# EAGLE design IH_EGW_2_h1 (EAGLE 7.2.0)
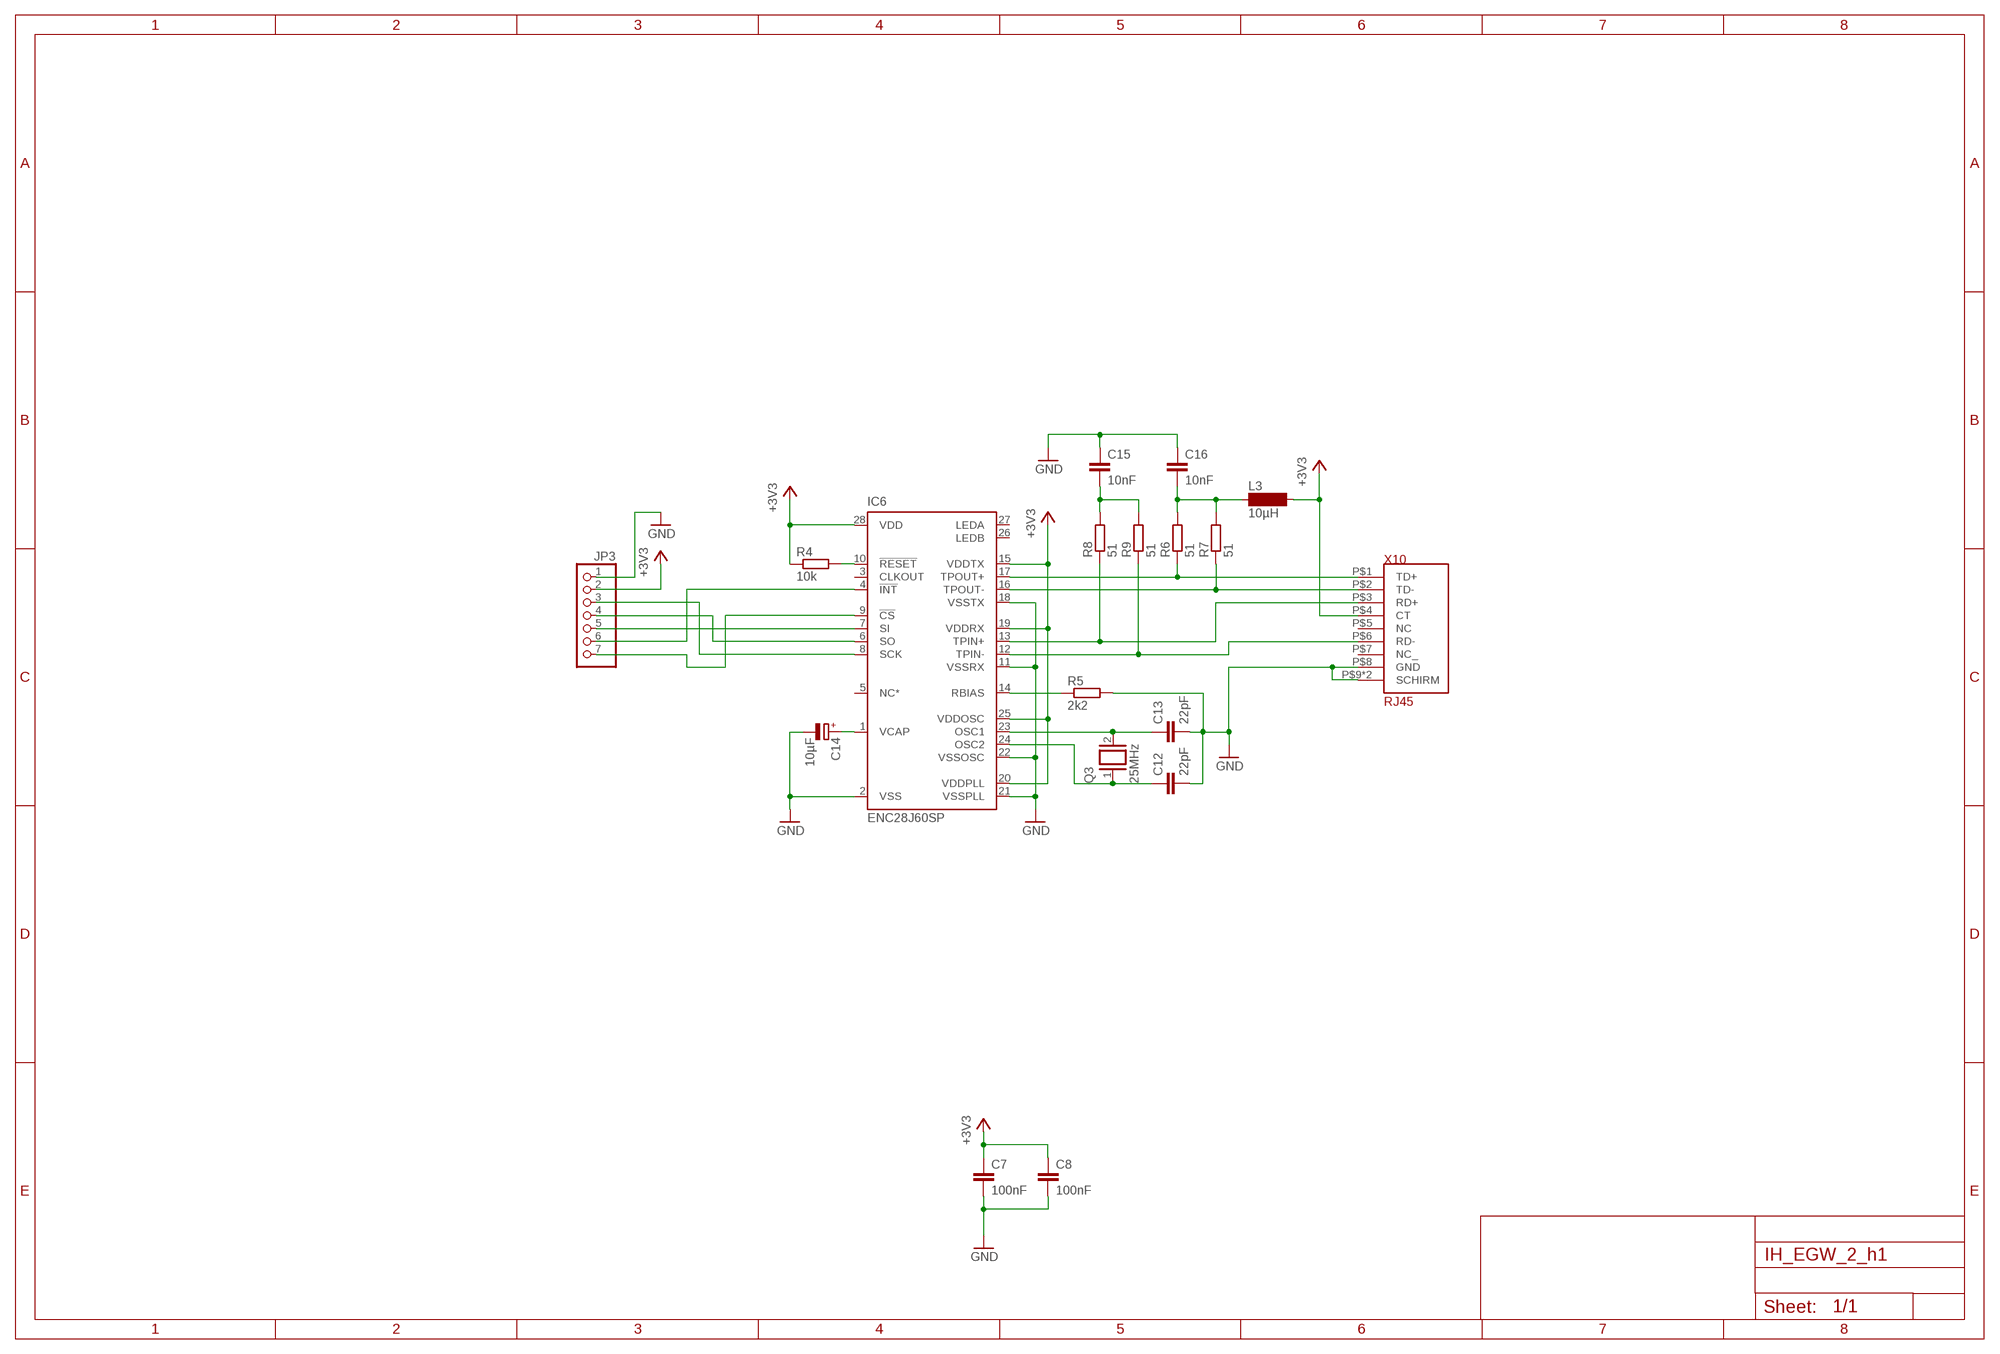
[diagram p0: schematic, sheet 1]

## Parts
C7  100nF  C-EUC0805  [C0805]
C8  100nF  C-EUC0805  [C0805]
C12  22pF  C-EUC0805  [C0805]
C13  22pF  C-EUC0805  [C0805]
C14  10µF  CPOL-EUE2-5  [E2-5]
C15  10nF  C-EUC0805  [C0805]
C16  10nF  C-EUC0805  [C0805]
IC6  ENC28J60SP  [DIL28-3]
JP3  PINHD-1X7  [1X07]
L3  10µH  SD12-1000  [SD12_1000]
Q3  25MHz  XTAL/S  [QS]
R4  10k  R-EU_R0805  [R0805]
R5  2k2  R-EU_R0805  [R0805]
R6  51  R-EU_M0805  [M0805]
R7  51  R-EU_M0805  [M0805]
R8  51  R-EU_M0805  [M0805]
R9  51  R-EU_M0805  [M0805]
X10  RJ45  [RJ45_LIEGEND]

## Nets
+3V3: C7.1 C8.1 IC6.15(VDDTX) IC6.19(VDDRX) IC6.20(VDDPLL) IC6.25(VDDOSC) IC6.28(VDD) JP3.2 L3.2 R4.1 X10.P$4(CT)
GND: C7.2 C8.2 C12.2 C13.2 C14.- C15.1 C16.1 IC6.2(VSS) IC6.11(VSSRX) IC6.18(VSSTX) IC6.21(VSSPLL) IC6.22(VSSOSC) JP3.1 R5.2 X10.P$8(GND) X10.P$9(SCHIRM) X10.P$10(SCHIRM)
INT_E: IC6.4(!INT) JP3.6
MISO: IC6.6(SO) JP3.4
N$1: IC6.7(SI) JP3.5
N$5: IC6.14(RBIAS) R5.1
N$6: C14.+ IC6.1(VCAP)
N$9: IC6.13(TPIN+) R8.1 X10.P$3(RD+)
N$10: IC6.12(TPIN-) R9.1 X10.P$6(RD-)
N$11: IC6.17(TPOUT+) R6.1 X10.P$1(TD+)
N$12: IC6.16(TPOUT-) R7.1 X10.P$2(TD-)
N$13: C15.2 R8.2 R9.2
N$14: C16.2 L3.1 R6.2 R7.2
N$28: C13.1 IC6.23(OSC1) Q3.2
N$29: C12.1 IC6.24(OSC2) Q3.1
N$30: IC6.10(!RESET) R4.2
SCK: IC6.8(SCK) JP3.3
SS: IC6.9(!CS) JP3.7
Unconnected: IC6.3(CLKOUT) IC6.5(NC*) IC6.26(LEDB) IC6.27(LEDA) X10.P$5(NC) X10.P$7(NC_)

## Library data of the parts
C7 C8 C12 C13 C15 C16 = rcl:C-EU: CAPACITOR, European symbol
C14 = rcl:CPOL-EU: POLARIZED CAPACITOR, European symbol
IC6 = microchip:ENC28J60: Stand-Alone Ethernet Controller with SPI Interface Source: http://ww1.microchip.com/downloads/en/DeviceDoc/39662c.pdf; MF: MICROCHIP; MPN: ENC28J60/SP; OC_FARNELL: 1084619; OC_NEWARK: 96K3661
JP3 = pinhead:PINHD-1X7: PIN HEADER
L3 = inductor-neosid:SD12: INDUCTOR; OC_FARNELL: unknown; OC_NEWARK: unknown
Q3 = special:XTAL/S: CRYSTAL
R4-R9 = resistor:R-EU_: RESISTOR, European symbol
X10 = RJ45:RJ45

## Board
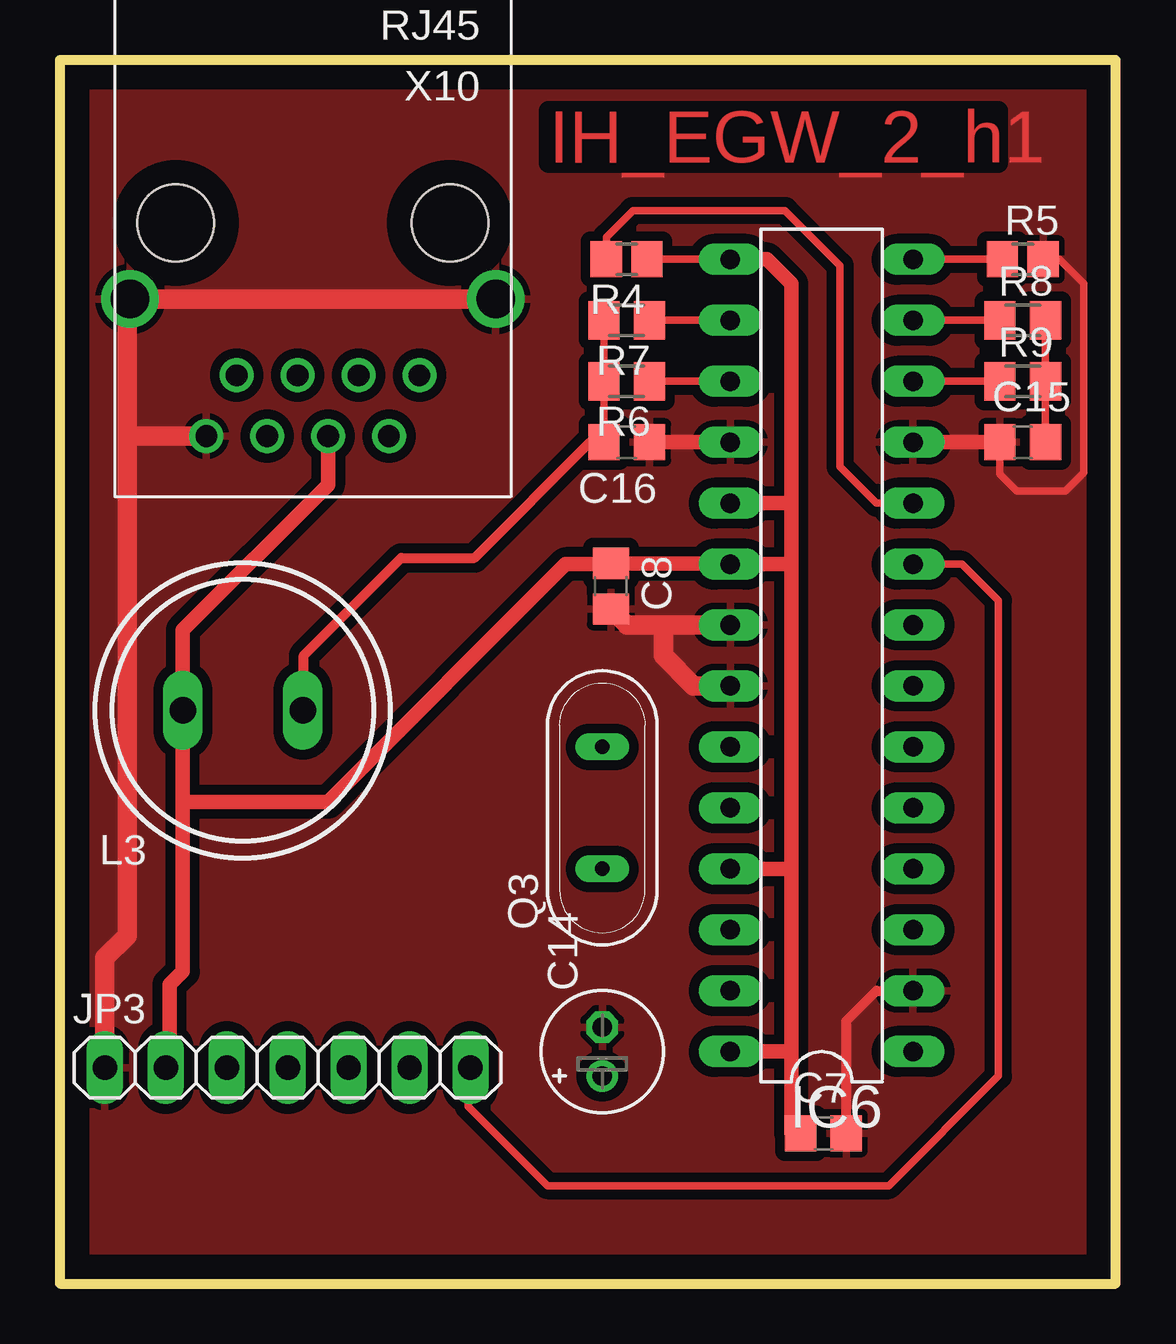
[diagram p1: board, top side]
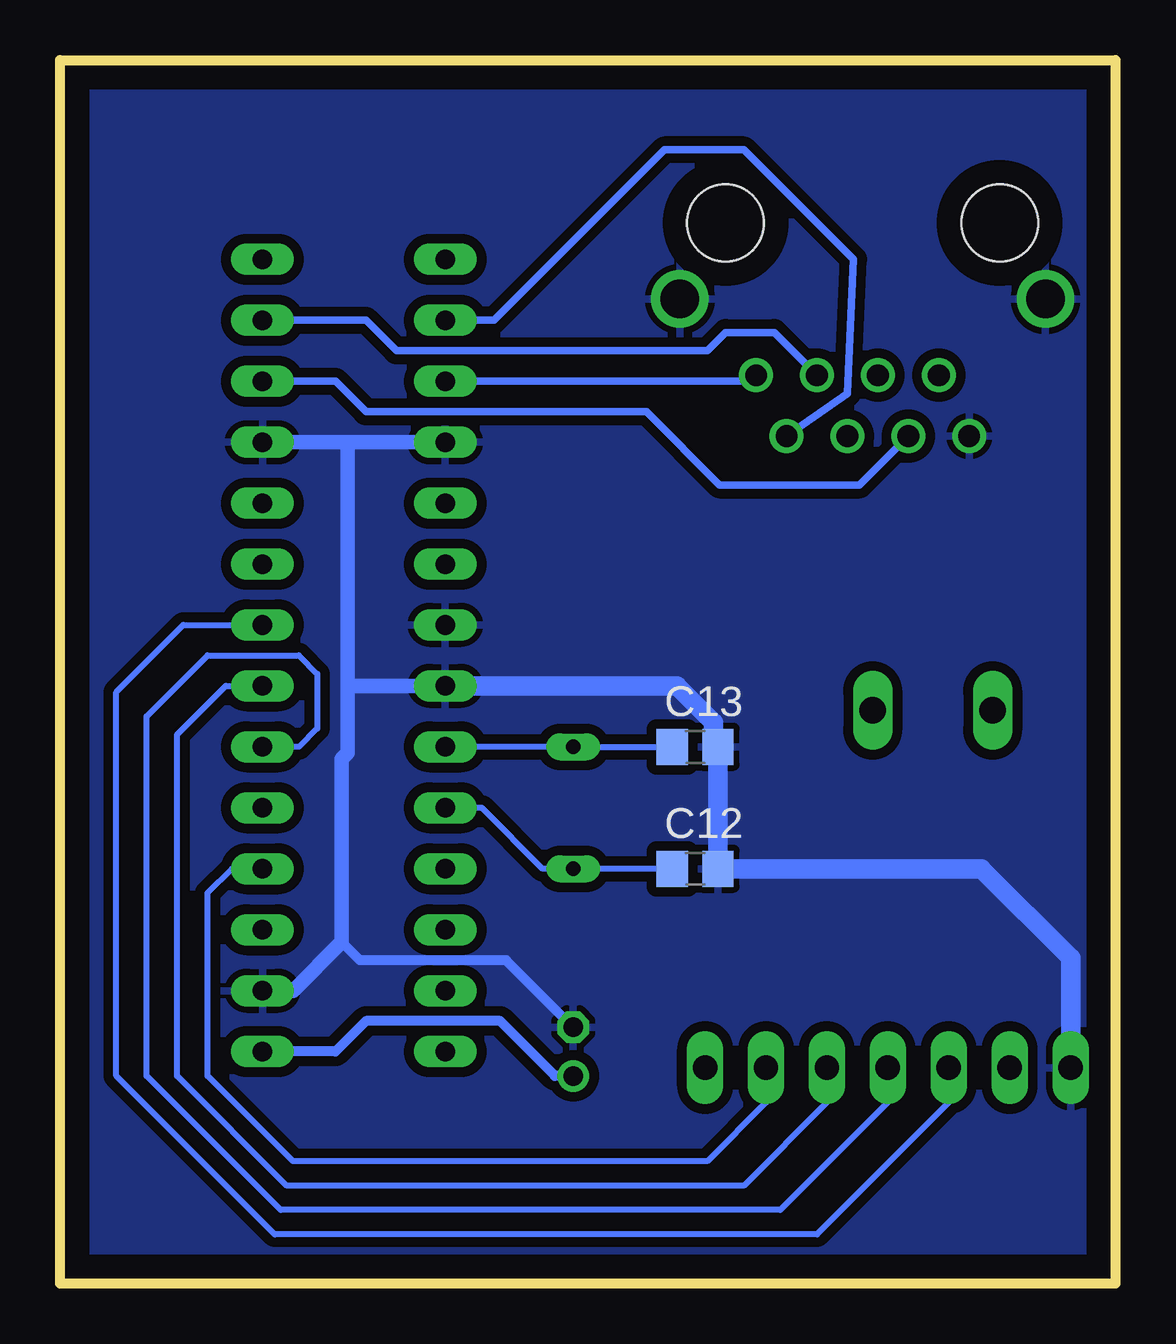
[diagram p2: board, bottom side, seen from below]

Size 44 x 51 mm. Coordinates in mm from the lower left corner, seen from the top.
Outline: 0,0 0,51 44,51 44,0 0,0
Copper layers (1*16): Top 0.035mm / dielectric 1.5mm / Bottom 0.035mm
Design rules "default *": minimum track width 10mil, minimum drill 36mil, track to track 15mil, track to pad 15mil, pad to pad 10mil, via to via 10mil, smd to smd 10mil, copper to edge 40mil, drill to drill 8mil, minimum pad ring 10mil, minimum via ring 8mil, stop-mask expansion 4mil, vias tented up to drill 0mil, thermal gap 10mil

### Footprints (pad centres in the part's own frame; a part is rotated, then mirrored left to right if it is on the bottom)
C0805 = smd 1.3 x 1.5: 1 -0.95,0; 2 0.95,0
E2-5 = drill 0.813 pad 1.27: + -1.016,0 | drill 0.813 pad 1.27 octagon: - 1.016,0
DIL28-3 = drill 0.813 long: 1 -16.51,-3.81; 2 -13.97,-3.81; 3 -11.43,-3.81; 4 -8.89,-3.81; 5 -6.35,-3.81; 6 -3.81,-3.81; 7 -1.27,-3.81; 8 1.27,-3.81; 9 3.81,-3.81; 10 6.35,-3.81; 11 8.89,-3.81; 12 11.43,-3.81; 13 13.97,-3.81; 14 16.51,-3.81; 15 16.51,3.81; 16 13.97,3.81; 17 11.43,3.81; 18 8.89,3.81; 19 6.35,3.81; 20 3.81,3.81; 21 1.27,3.81; 22 -1.27,3.81; 23 -3.81,3.81; 24 -6.35,3.81; 25 -8.89,3.81; 26 -11.43,3.81; 27 -13.97,3.81; 28 -16.51,3.81
1X07 = drill 1.016 long: 1 -7.62,0; 2 -5.08,0; 3 -2.54,0; 4 0,0; 5 2.54,0; 6 5.08,0; 7 7.62,0
SD12_1000 = drill 1.1 long: 1 -2.5,0; 2 2.5,0
QS = drill 0.61 long: 1 -2.54,0; 2 2.54,0
R0805 = smd 1.3 x 1.5: 1 -0.85,0; 2 0.85,0
M0805 = smd 1.3 x 1.6: 1 -0.95,0; 2 0.95,0
RJ45_LIEGEND = drill 0.9: P$1 2.54,1.27; P$2 3.81,3.81; P$3 5.08,1.27; P$4 6.35,3.81; P$5 7.62,1.27; P$6 8.89,3.81; P$7 10.16,1.27; P$8 11.43,3.81 | drill 1.6: P$9 -0.635,-1.905; P$10 14.605,-1.905 | hole 3.2: 1.27,-5.08; 12.7,-5.08

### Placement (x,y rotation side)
C7  31.82,6.26 0 top
C8  22.96,29.07 270 top
C12  17.53,17.29 0 bottom
C13  17.53,22.37 0 bottom
C14  22.61,9.67 90 top
C15  40.13,35.07 0 top
C16  23.62,35.07 180 top
IC6  31.75,26.18 90 top
JP3  9.49,9 0 top
L3  7.62,23.89 180 top
Q3  22.61,19.83 90 top
R4  23.62,42.69 180 top
R5  40.13,42.69 0 top
R6  23.62,37.61 180 top
R7  23.62,40.15 180 top
R8  40.13,40.15 0 top
R9  40.13,37.61 0 top
X10  17.53,39.13 180 top

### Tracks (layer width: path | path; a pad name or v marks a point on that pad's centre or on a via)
+3V3
  Top 0.305: R4.1 IC6.15
  Top 0.61: 30.48,29.99 IC6.20 27.91,30.02 C8.1 22.93,29.99 21.08,29.99 11.18,20.08 5.12,20.08 | 30.48,29.99 30.48,32.53 | 30.48,32.53 30.48,41.67 29.46,42.69 IC6.15 | IC6.19 30.48,32.53 | IC6.28 30.48,9.67 | 30.48,9.67 30.48,17.29 | 30.48,17.29 30.48,29.99 | IC6.25 30.48,17.29 | C7.1 30.48,6.26 30.48,9.67 | JP3.2 4.57,9.16 4.57,12.46 5.12,13.01 5.12,20.08 | 5.12,20.08 L3.2 5.12,27.23 11.18,33.29 X10.P$4
GND
  Top 0.305: R5.2 41.66,42.69 42.67,41.67 42.67,33.8 41.91,33.04 39.88,33.04 39.18,33.73 C15.1
  Top 0.406: C7.2 32.77,10.95 34.04,12.21 IC6.2
  Top 0.61: IC6.11 C15.1 | C16.1 IC6.18
  Top 0.813: X10.P$9 X10.P$10 2.79,40.91 2.79,35.58 | 2.79,35.58 2.79,14.49 1.87,13.57 JP3.1 | X10.P$8 3.05,35.32 2.79,35.58 | C8.2 23.63,27.45 25.15,27.45 | 25.15,27.45 IC6.21 | IC6.22 26.42,24.91 25.15,26.18 25.15,27.45
  Bottom 0.406: 32.26,14.24 31.5,13.48 25.4,13.48 C14.-
  Bottom 0.61: IC6.11 32,35.07 | 32,35.07 IC6.18 | IC6.2 34.29,12.21 32.26,14.24 32.26,21.86 32,22.11 32,24.91 | 32,24.91 32,35.07 | IC6.22 32,24.91
  Bottom 0.813: JP3.1 1.87,13.57 5.59,17.29 C12.2 C13.2 16.76,22.56 16.76,23.38 18.29,24.91 IC6.22
  pour Bottom (isolate 0.406): -1.52,51.83 -1.52,-1 45.97,-1 45.97,51.83
  pour Top (isolate 0.406): -1.27,52.09 -1.27,-1.51 45.97,-1.51 45.97,52.34 -1.52,52.34
INT_E
  Bottom 0.254: JP3.6 14.57,7.54 17.02,5.1 34.29,5.1 37.85,8.65 37.85,16.27 36.83,17.29 IC6.4
MISO
  Bottom 0.254: JP3.4 9.49,7.54 13.97,3.06 34.8,3.06 40.39,8.65 40.39,23.64 37.85,26.18 34.04,26.18 33.27,25.42 33.27,23.13 34.04,22.37 IC6.6
N$1
  Bottom 0.254: JP3.5 12.03,7.54 15.49,4.08 34.54,4.08 39.12,8.65 39.12,22.88 37.08,24.91 IC6.7
N$5
  Top 0.305: IC6.14 R5.1
N$6
  Bottom 0.406: C14.+ 23.37,8.65 25.65,10.94 31.24,10.94 32.51,9.67 IC6.1
N$9
  Top 0.305: IC6.13 R8.1
  Bottom 0.305: IC6.13 31.24,40.15 29.97,38.88 17.02,38.88 16.26,39.64 14.22,39.64 X10.P$3
N$10
  Top 0.305: IC6.12 R9.1
  Bottom 0.305: IC6.12 32.51,37.61 31.24,36.34 19.56,36.34 16.51,33.29 10.67,33.29 X10.P$6
N$11
  Top 0.305: R6.1 IC6.17
  Bottom 0.305: X10.P$1 15.24,37.61 IC6.17
N$12
  Top 0.305: R7.1 IC6.16
  Bottom 0.305: IC6.16 25.91,40.15 18.8,47.26 15.49,47.26 10.92,42.69 11.18,37.1 X10.P$2
N$13
  Top 0.305: R8.2 R9.2 C15.2
N$14
  Top 0.305: R7.2 R6.2 C16.2
  Top 0.406: L3.1 10.16,23.93 10.16,26.18 14.22,30.24 17.27,30.24 22.1,35.07 C16.2
N$28
  Bottom 0.254: IC6.23 Q3.2 C13.1
N$29
  Bottom 0.254: C12.1 Q3.1 23.88,17.29 26.42,19.83 IC6.24
N$30
  Top 0.305: R4.2 22.77,43.62 23.88,44.72 30.23,44.72 32.51,42.43 32.51,34.05 34.04,32.53 IC6.10
SCK
  Bottom 0.254: JP3.3 6.95,7.54 12.45,2.05 35.05,2.05 41.66,8.65 41.66,24.65 38.86,27.45 IC6.8
SS
  Top 0.305: JP3.7 17.02,8.91 17.02,7.38 20.32,4.08 34.54,4.08 39.12,8.65 39.12,28.46 37.59,29.99 IC6.9

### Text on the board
Top: IH_EGW_2_h1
